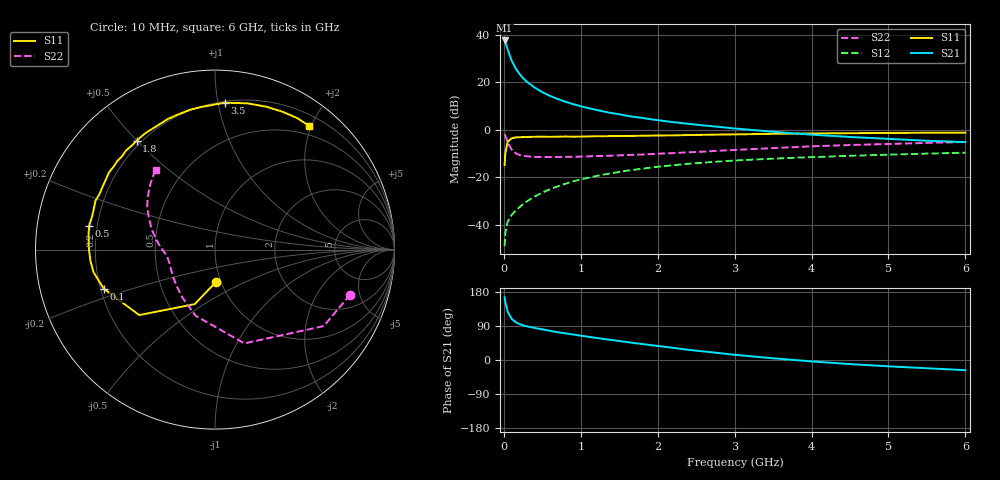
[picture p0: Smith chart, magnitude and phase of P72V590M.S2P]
! SIEMENS Small Signal Semiconductors
! BFP196
! Si NPN RF Bipolar Junction Transistor in SOT143
! VCE = 2.5 V  IC = 90 mA
! Common Emitter S-Parameters:  May  1996
# GHz  S  MA  R  50
!  f  S11  S21  S12  S22
! GHz  MAG  ANG  MAG  ANG  MAG  ANG  MAG  ANG
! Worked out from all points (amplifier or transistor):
!   36 points, 10 MHz to 6 GHz, reference 50 ohm
!   highest |S21| = 37.7 dB at 10 MHz (marker M1)
!   |S21| within 3 dB of that: start of sweep to 41.76 MHz
!   unconditionally stable (mu >= 1): 306.7 MHz to 4.819 GHz
!   at 250 MHz: K = 0.96, MSG = 26.6 dB, |S12| = -31.4 dB
!   at 1.4 GHz: K = 1.10, MAG = 10.8 dB, |S12| = -18.4 dB
!   at 6 GHz: K = 0.99, MSG = 2.2 dB, |S12| = -9.7 dB
!   S11 on the Smith chart (normalised r, x): 10 MHz: 0.95, -0.35; 100 MHz: 0.21, -0.16; 500 MHz: 0.17, +0.09; 1.8 GHz: 0.18, +0.50; 3.5 GHz: 0.21, +1.04; 6 GHz: 0.36, +1.97
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0.01  0.1804 -88.4  76.5 165.8  0.0035 74.1  0.7939 -18.4
0.02  0.3243 -110.4  70.13 152.3  0.0067 64.9  0.7407 -35.1
0.05  0.5582 -139.2  49.11 127.1  0.0116 54.3  0.5476 -72.6
0.1  0.6566 -160.6  29 108.8  0.0158 52.6  0.384 -106.3
0.15  0.6883 -169.4  20.11 100.4  0.0195 55.3  0.3226 -124.5
0.2  0.6967 -174.7  15.31 95.1  0.0229 58.8  0.2954 -135.8
0.25  0.7008 -178.9  12.25 91.5  0.027 61.0  0.2821 -144.1
0.3  0.7041 178.3  10.27 88.9  0.0309 62.5  0.2753 -149.2
0.4  0.7099 172.7  7.76 84.5  0.039 65.6  0.2678 -156.7
0.5  0.7137 169.2  6.207 80.8  0.0473 66.1  0.2651 -161.4
0.6  0.709 164.7  5.176 77.0  0.0557 66.6  0.2649 -164.8
0.7  0.713 161.0  4.453 73.3  0.064 66.4  0.2658 -167.3
0.9  0.7141 154.3  3.471 67.3  0.0814 64.4  0.2685 -171.1
1.1  0.7229 147.3  2.853 61.2  0.0974 62.3  0.2748 -173.8
1.4  0.7349 137.8  2.249 52.9  0.1209 58.1  0.2843 -177.4
1.8  0.7477 125.7  1.772 42.2  0.1511 51.8  0.3 178.0
2.2  0.7607 115.4  1.448 32.1  0.1787 45.7  0.3214 172.7
2.8  0.7914 100.1  1.148 18.2  0.2139 36.5  0.3618 163.9
3.5  0.8202 86.3  0.906 4.5  0.246 26.3  0.4105 154.1
4.5  0.8457 70.3  0.704 -10.8  0.2825 14.1  0.476 141.9
5.5  0.8639 58.1  0.586 -21.8  0.3139 3.3  0.5281 131.7
6  0.8661 52.6  0.548 -26.8  0.3287 -2.5  0.553 126.7
